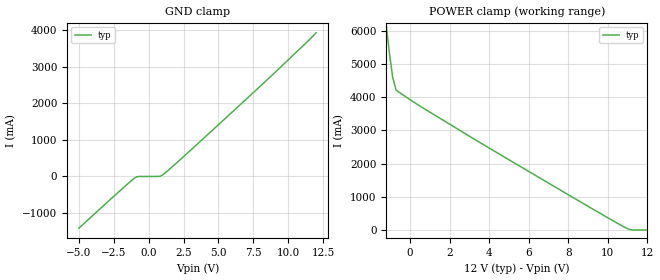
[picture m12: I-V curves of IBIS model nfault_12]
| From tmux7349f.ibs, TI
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| nfault_12
[Model]   nfault_12
Model_type   Input
Vinl = 0.8
Vinh = 1.3
|   typ   min   max
C_comp   1.598234e-11   NA   NA
[Voltage Range]   12   NA   NA
[Temperature Range]   27   NA   NA
[Power Clamp Reference]   12   NA   NA
[GND Clamp Reference]   0   NA   NA
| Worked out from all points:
|   GND clamp passes 1 mA (typ) near -0.72 V on its own axis
[GND Clamp]
|   Voltage   I(typ)   I(min)   I(max)
-5V       -1.413A    NA         NA
-1.737V   -280.9mA   NA         NA
-878.8mV  -12.23mA   NA         NA
838.4mV   6.24mA     NA         NA
1.182V    96.25mA    NA         NA
8.394V    2.607A     NA         NA
12V       3.924A     NA         NA
[POWER Clamp]
|   Voltage   I(typ)   I(min)   I(max)
-5V       31.98A     NA         NA
-1.222V   6.271A     NA         NA
-1.05V    5.373A     NA         NA
-878.8mV  4.604A     NA         NA
-707.1mV  4.216A     NA         NA
-535.4mV  4.138A     NA         NA
494.9mV   3.733A     NA         NA
3.586V    2.614A     NA         NA
10.63V    158.7mA    NA         NA
11.14V    8.913mA    NA         NA
12V       -7.614uA   NA         NA
